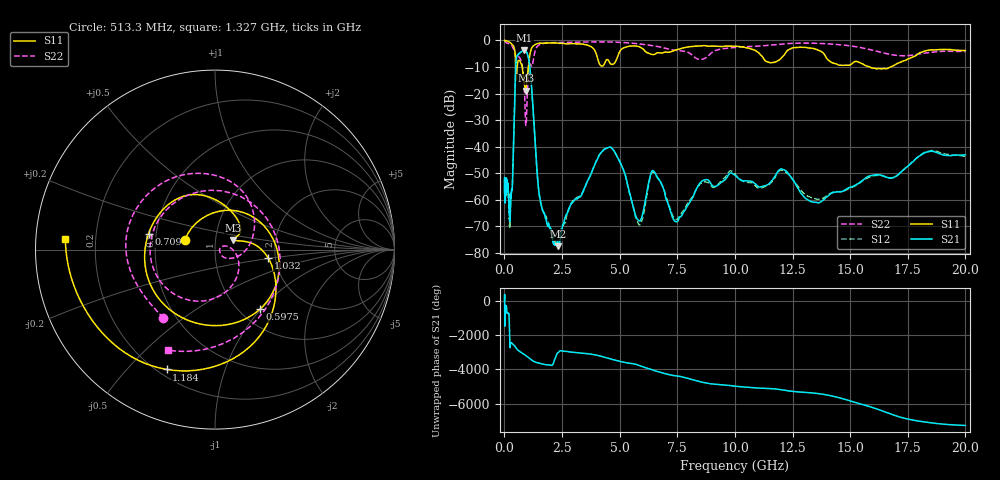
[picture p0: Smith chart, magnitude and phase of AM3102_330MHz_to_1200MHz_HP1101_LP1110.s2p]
! Date/Time: Tue, Sep 11, 2018 5:22 PM
! Network Analyzer: Agilent Technologies E8362B Rev: A.07.50.63
! Sweep from 0.010 to 20.000 GHz, 1601 Points, Sweep Type: LOG
! Power Supply: 4.949 V, 0.001 A
# Hz S DB R 50
!freq MagS11 AngS11 MagS21 AngS21 MagS12 AngS12 MagS22 AngS22
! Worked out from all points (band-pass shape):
!   1601 points, 10 MHz to 20 GHz, reference 50 ohm
!   highest |S21| = -3.68 dB at 869.7 MHz (marker M1); lowest = -77.5 dB at 2.325 GHz (marker M2)
!   |S21| within 3 dB of the highest: 522.1 MHz to 1.047 GHz (524.8 MHz wide, 66.9 % of centre)
!   lowest |S11| = -18.9 dB at 925.1 MHz (marker M3), VSWR 1.26, Z = 60.8 + j6.54 ohm
!   |S11| at or under -10 dB: 486.4 MHz to 555 MHz (68.61 MHz wide, 13.2 % of centre); 771.9 MHz to 1.037 GHz (265.5 MHz wide, 29.3 % of centre); 15.86 GHz to 16.75 GHz (891.9 MHz wide, 5.47 % of centre)
!   |S22| runs from -32.0 to -0.2 dB; largest |S21 - S12| = 0.0096
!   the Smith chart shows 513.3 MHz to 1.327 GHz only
!   S11 on the Smith chart (normalised r, x): 513.3 MHz: 0.71, +0.08; 597.5 MHz: 1.23, -0.99; 709 MHz: 0.45, +0.09; 1.032 GHz: 1.83, -0.19; 1.184 GHz: 0.23, -0.65; 1.327 GHz: 0.09, +0.04
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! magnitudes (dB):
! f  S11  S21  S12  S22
! 10 MHz  0.0  -53.2  -53.8  -0.3
! 35.55 MHz  -0.1  -58.3  -59.3  -0.5
! 126.4 MHz  -0.2  -54.0  -54.2  -1.0
! 241.2 MHz  -0.7  -66.7  -69.5  -1.4
! 351 MHz  -1.6  -54.0  -53.8  -2.4
! 447.2 MHz  -3.6  -21.6  -21.6  -4.2
! 513.3 MHz  -15.1  -7.3  -7.4  -6.4
! 597.5 MHz  -7.6  -5.3  -5.4  -6.0
! 709 MHz  -8.4  -4.4  -4.4  -7.3
! 869.7 MHz  -15.9  -3.7  -3.7  -18.5
! 925.1 MHz  -18.9  -3.9  -4.0  -31.7
! 1.032 GHz  -10.4  -6.1  -6.1  -13.9
! 1.184 GHz  -2.9  -18.0  -17.9  -9.7
! 1.327 GHz  -1.6  -37.6  -38.0  -4.2
! 1.59 GHz  -1.0  -61.5  -61.8  -1.3
! 2.325 GHz  -1.0  -77.5  -75.6  -0.8
! 4.457 GHz  -7.2  -40.5  -40.4  -0.5
! 5.652 GHz  -2.1  -64.7  -65.1  -1.1
! 6.518 GHz  -5.2  -49.6  -50.1  -2.1
! 7.517 GHz  -3.4  -68.1  -67.2  -3.8
! 8.627 GHz  -2.0  -52.7  -53.3  -7.0
! 20 GHz  -3.8  -43.1  -43.6  -4.2
